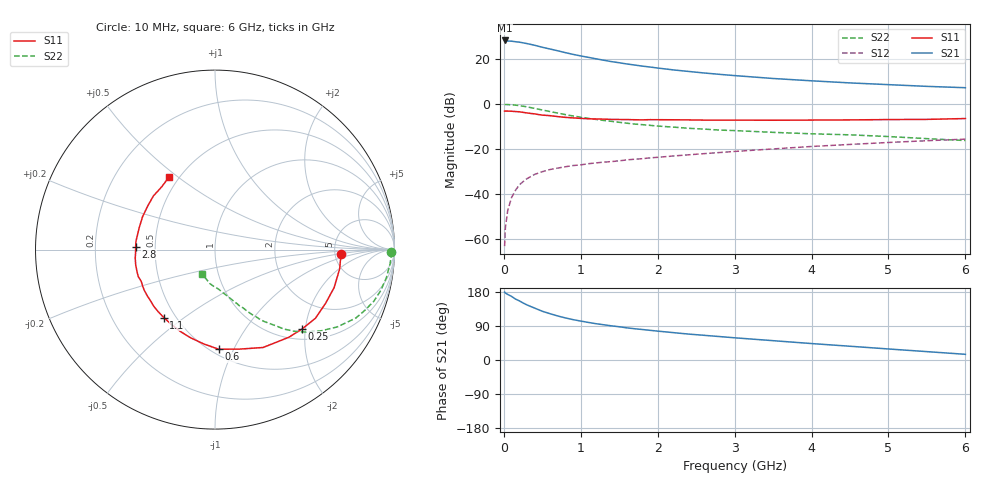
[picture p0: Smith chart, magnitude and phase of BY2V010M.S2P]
! SIEMENS Small Signal Semiconductors
! BFY420
! Si NPN RF SIEGET Grounded Emitter Transistor in MICRO-X
! VCE = 2 V  IC = 10 mA
! Common Emitter S-Parameters:  October  1996
# GHz  S  MA  R  50
!  f  S11  S21  S12  S22
! GHz  MAG  ANG  MAG  ANG  MAG  ANG  MAG  ANG
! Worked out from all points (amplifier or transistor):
!   36 points, 10 MHz to 6 GHz, reference 50 ohm
!   highest |S21| = 28.3 dB at 10 MHz (marker M1)
!   |S21| within 3 dB of that: start of sweep to 497 MHz
!   unconditionally stable (mu >= 1): 2.494 GHz to end of sweep
!   at 250 MHz: K = 0.19, MSG = 30.8 dB, |S12| = -34.4 dB
!   at 1.4 GHz: K = 0.75, MSG = 22.2 dB, |S12| = -25.5 dB
!   at 6 GHz: K = 1.10, MAG = 9.5 dB, |S12| = -15.5 dB
!   S11 on the Smith chart (normalised r, x): 10 MHz: 5.68, -0.58; 250 MHz: 1.23, -1.92; 600 MHz: 0.55, -0.88; 1.1 GHz: 0.43, -0.42; 2.8 GHz: 0.39, +0.02; 6 GHz: 0.44, +0.47
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0.01  0.7034 -2.1  26.03 179.2  0.0007 98.5  0.9805 -0.8
0.02  0.7017 -3.7  25.91 176.7  0.0018 89.3  0.9827 -1.7
0.1  0.6967 -17.7  25.06 167.9  0.0084 81.0  0.9678 -9.3
0.15  0.6851 -25.9  24.44 161.0  0.0121 79.0  0.951 -13.9
0.2  0.6778 -34.4  23.89 156.2  0.016 75.1  0.9306 -18.0
0.25  0.6565 -42.4  23.05 150.5  0.019 69.9  0.9005 -22.1
0.3  0.6385 -49.9  22.2 145.4  0.0221 68.2  0.8726 -25.9
0.4  0.6077 -63.8  20.37 137.0  0.0275 62.7  0.8061 -32.3
0.5  0.5712 -76.1  18.37 128.6  0.0316 58.2  0.7425 -37.6
0.6  0.5554 -87.8  16.81 122.2  0.0353 55.8  0.6854 -42.1
0.7  0.5297 -96.7  15.36 116.2  0.038 53.6  0.6336 -45.9
0.8  0.5093 -105.7  13.95 111.1  0.0407 51.0  0.5868 -49.0
0.9  0.4953 -112.9  12.77 106.5  0.0433 49.8  0.5467 -51.2
1.1  0.474 -127.0  10.96 99.1  0.0476 49.3  0.4843 -55.7
1.3  0.4652 -136.9  9.461 92.9  0.0517 48.2  0.4342 -58.8
1.6  0.4546 -150.1  7.816 84.8  0.0579 47.5  0.3773 -63.1
2.2  0.4502 -168.8  5.783 72.3  0.0705 46.5  0.3098 -69.7
2.8  0.4424 177.9  4.606 61.9  0.0841 45.0  0.2658 -75.2
3.5  0.4395 163.7  3.72 51.0  0.1012 42.0  0.2364 -81.2
4.5  0.4469 146.8  2.967 36.3  0.1275 35.7  0.2082 -90.7
5.5  0.4594 130.0  2.486 22.1  0.1543 27.7  0.1714 -106.3
6  0.4792 122.2  2.321 15.0  0.1671 23.4  0.1556 -117.0
